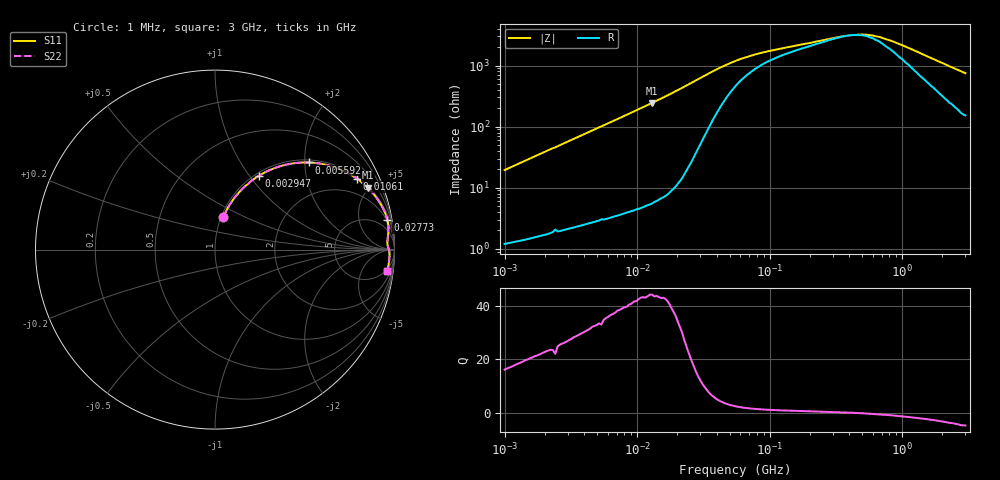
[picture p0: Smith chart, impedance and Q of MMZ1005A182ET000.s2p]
! S-parameter Generated by TDK Corporation
! Copyright(C) 2016 TDK Corporation.
! All Rights Reserved.
! TDK P/N: MMZ1005A182ET000 (Chip Beads)
! Property: |Z|=1800¶ at 100MHz
! Size(LxWxT): 1x0.5x0.5mm, 0.039x0.02x0.02inches
! Model Type: s2p (Touchstone File Format Version 1.0)
! Frequency: DC=Yes Start=1MHz Stop=3000MHz 202points Log-sweep
! Note: This model was converted from impedance.
! Model Generated on May. 16, 2016
! Hash(MD5):
! Port Assignments:
!  1 ---@@@--- 2
! Applicable Conditions:
!  Temperature = 25 degC
!  DC Bias Current = 0 A
!  Small Signal Operation
! Terms and conditions regarding TDK Simulation Models
! (1)This simulation model is being provided solely for informational purposes. Please refer to the specifications of the products in terms of detailed characteristics of such products.
! (2)In no event shall TDK Corporation of any of its subsidiaries be liable for any loss or damage arising, directly or indirectly,
!  From any information contained in this simulation model, including, but not limited to loss or damages arising from any inaccuracies, omissions or errors in connection with such information.
! (3)Any and all copyrights on this simulation model are owned by TDK Corporation.
!  Duplication or redistribution of this simulation model without prior written permission from TDK Corporation is prohibited.
! (4)This simulation model is subject to any modification or change without any prior notice.
! (5)Neither TDK Corporation nor any of its subsidiaries shall make any warranty, express or implied,
!  Including but not limited to the correctness, implied warranties of merchantability and fitness for a particular purpose with respect to this simulation models.
! (6)The use of this simulation model shall be deemed to have consented to the terms and conditions hereof.
# MHz S MA R 50
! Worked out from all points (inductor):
!   201 points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, 1 MHz to 3 GHz, reference 50 ohm
!   read as one part in series: L = 3.08 uH near 1.041 MHz
!   highest Q = 43.8 at 12.96 MHz (marker M1), where L = 3 uH
!   self-resonance near 406.9 MHz
!   S11 on the Smith chart (normalised r, x): 1 MHz: 1.02, +0.39; 2.947 MHz: 1.04, +1.12; 5.592 MHz: 1.06, +2.10; 10.61 MHz: 1.09, +3.98; 27.73 MHz: 2, +11; 3 GHz: 4, -15
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1  0.1887 75.6  0.9705 -10.9  0.9705 -10.9  0.1887 75.6
1.751453  0.3151 69.0  0.9345 -18.3  0.9345 -18.3  0.3151 69.0
2.412589  0.4089 63.3  0.8943 -24.1  0.8943 -24.1  0.4089 63.3
2.947212  0.481 59.1  0.859 -28.7  0.859 -28.7  0.481 59.1
3.900413  0.584 52.4  0.7926 -35.7  0.7926 -35.7  0.584 52.4
5.592179  0.7135 42.9  0.6804 -45.5  0.6804 -45.5  0.7135 42.9
7.400828  0.8008 35.3  0.5785 -53.2  0.5785 -53.2  0.8008 35.3
10.61086  0.8852 26.4  0.4451 -62.2  0.4451 -62.2  0.8852 26.4
12.9622  0.9181 22.1  0.3761 -66.6  0.3761 -66.6  0.9181 22.1
14.61624  0.9337 19.7  0.3372 -69.0  0.3372 -69.0  0.9337 19.7
20.13356  0.9624 14.2  0.2451 -74.2  0.2451 -74.2  0.9624 14.2
27.73354  0.9744 9.8  0.1708 -76.5  0.1708 -76.5  0.9744 9.8
41.38676  0.9715 6.0  0.1076 -71.7  0.1076 -71.7  0.9715 6.0
54.77226  0.966 4.3  0.08168 -63.2  0.08168 -63.2  0.966 4.3
88.54986  0.9613 2.6  0.05878 -47.5  0.05878 -47.5  0.9613 2.6
213.6344  0.9638 1.0  0.03997 -24.6  0.03997 -24.6  0.9638 1.0
359.4878  0.9682 0.2  0.03203 -6.2  0.03203 -6.2  0.9682 0.2
495.1867  0.9706 -0.4  0.03009 12.2  0.03009 12.2  0.9706 -0.4
682.1091  0.9722 -1.1  0.03328 32.8  0.03328 32.8  0.9722 -1.1
800.5644  0.9725 -1.5  0.03742 41.9  0.03742 41.9  0.9725 -1.5
1645.649  0.9721 -3.9  0.07281 65.5  0.07281 65.5  0.9721 -3.9
3000  0.9658 -7.2  0.1289 71.0  0.1289 71.0  0.9658 -7.2
